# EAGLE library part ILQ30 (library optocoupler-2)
SIEMENS OPTO COUPLER
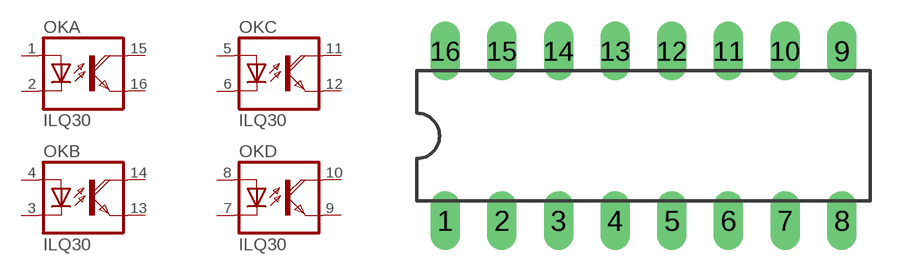
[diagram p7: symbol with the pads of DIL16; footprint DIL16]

Designator prefix OK; gates A=OK-D B=OK-D C=OK-D D=OK-D

## ILQ30  [DIL16]
1  A:A  pas
2  A:C  pas
3  B:C  pas
4  B:A  pas
5  C:A  pas
6  C:C  pas
7  D:C  pas
8  D:A  pas
9  D:EMI  pas
10  D:COL  pas
11  C:COL  pas
12  C:EMI  pas
13  B:EMI  pas
14  B:COL  pas
15  A:COL  pas
16  A:EMI  pas

## Footprint DIL16 (pad centres in mm)
Dual In Line Package
drill 0.813 long: 1 -8.89,-3.81; 2 -6.35,-3.81; 3 -3.81,-3.81; 4 -1.27,-3.81; 5 1.27,-3.81; 6 3.81,-3.81; 7 6.35,-3.81; 8 8.89,-3.81; 9 8.89,3.81; 10 6.35,3.81; 11 3.81,3.81; 12 1.27,3.81; 13 -1.27,3.81; 14 -3.81,3.81; 15 -6.35,3.81; 16 -8.89,3.81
